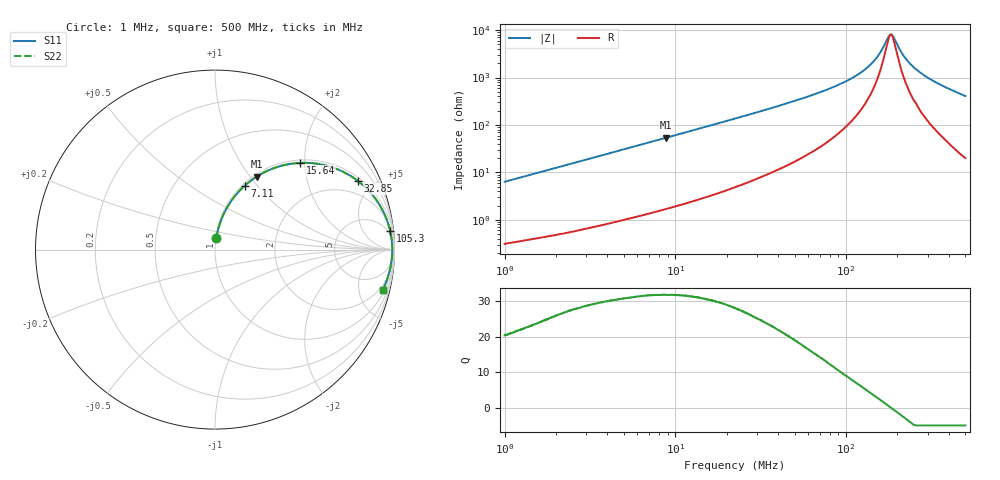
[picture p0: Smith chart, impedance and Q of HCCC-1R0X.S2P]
!s-Parameter Generated by FASTRON Sdn. Bhd.
!FASTRON P/N : HCCC-1R0X
!Keysight Technologies,E4991B,MY54100416,A.01.15
!Date: Thu Apr 02 13:34:52 2026
!Version  : Rev00 Thu Apr 02 13:34:52 2026
!Data & Calibration Information:
!PortZ  Port1:50+j0  Port2:50+j0
!When reading, reference impedance value at option line is always used.
! Remarks : This data is being provided solely for informational purposes.
!Freq	S11	S21	S12	S22
# Hz S dB R 50
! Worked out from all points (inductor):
!   1601 points, 1 MHz to 500 MHz, reference 50 ohm
!   read as one part in series: L = 1 uH near 1.032 MHz
!   highest Q = 31.8 at 8.837 MHz (marker M1), where L = 970 nH
!   self-resonance near 183.2 MHz
!   S11 on the Smith chart (normalised r, x): 1 MHz: 1.01, +0.13; 7.11 MHz: 1.03, +0.87; 15.64 MHz: 1.06, +1.90; 32.85 MHz: 1.17, +4.05; 105.3 MHz: 3, +18; 500 MHz: 1.40, -8.14
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1000000  -24.00 83.6  -0.04 -3.6  -0.04 -3.6  -24.00 83.6
2820919  -15.33 78.1  -0.18 -9.9  -0.18 -9.9  -15.33 78.1
4673927  -11.25 72.2  -0.42 -15.9  -0.42 -15.9  -11.25 72.2
7109882  -8.09 65.0  -0.85 -23.2  -0.85 -23.2  -8.09 65.0
7957584  -7.30 62.6  -1.03 -25.6  -1.03 -25.6  -7.30 62.6
8837438  -6.59 60.3  -1.22 -27.9  -1.22 -27.9  -6.59 60.3
1.564207e7  -3.38 45.5  -2.94 -42.7  -2.94 -42.7  -3.38 45.5
2.236068e7  -2.02 35.5  -4.70 -52.4  -4.70 -52.4  -2.02 35.5
3.28461e7  -1.09 25.8  -7.22 -61.9  -7.22 -61.9  -1.09 25.8
6.307767e7  -0.36 13.1  -12.90 -73.3  -12.90 -73.3  -0.36 13.1
1.053272e8  -0.16 6.1  -19.44 -77.0  -19.44 -77.0  -0.16 6.1
1.254438e8  -0.13 4.1  -22.83 -75.9  -22.83 -75.9  -0.13 4.1
1.437107e8  -0.12 2.6  -26.60 -72.0  -26.60 -72.0  -0.12 2.6
1.583655e8  -0.11 1.5  -30.55 -64.0  -30.55 -64.0  -0.11 1.5
1.77937e8  -0.11 0.3  -37.51 -23.4  -37.51 -23.4  -0.11 0.3
1.828413e8  -0.11 0.0  -38.26 -1.7  -38.26 -1.7  -0.11 0.0
1.878807e8  -0.11 -0.3  -37.65 20.9  -37.65 20.9  -0.11 -0.3
2.220328e8  -0.11 -2.1  -28.35 69.4  -28.35 69.4  -0.11 -2.1
2.437259e8  -0.12 -3.1  -25.05 74.3  -25.05 74.3  -0.12 -3.1
2.696248e8  -0.13 -4.3  -22.42 76.5  -22.42 76.5  -0.13 -4.3
3.497673e8  -0.18 -7.7  -17.47 77.2  -17.47 77.2  -0.18 -7.7
5e8  -0.35 -13.6  -12.55 73.6  -12.55 73.6  -0.35 -13.6
